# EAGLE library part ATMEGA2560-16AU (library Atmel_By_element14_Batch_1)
Microcontroller
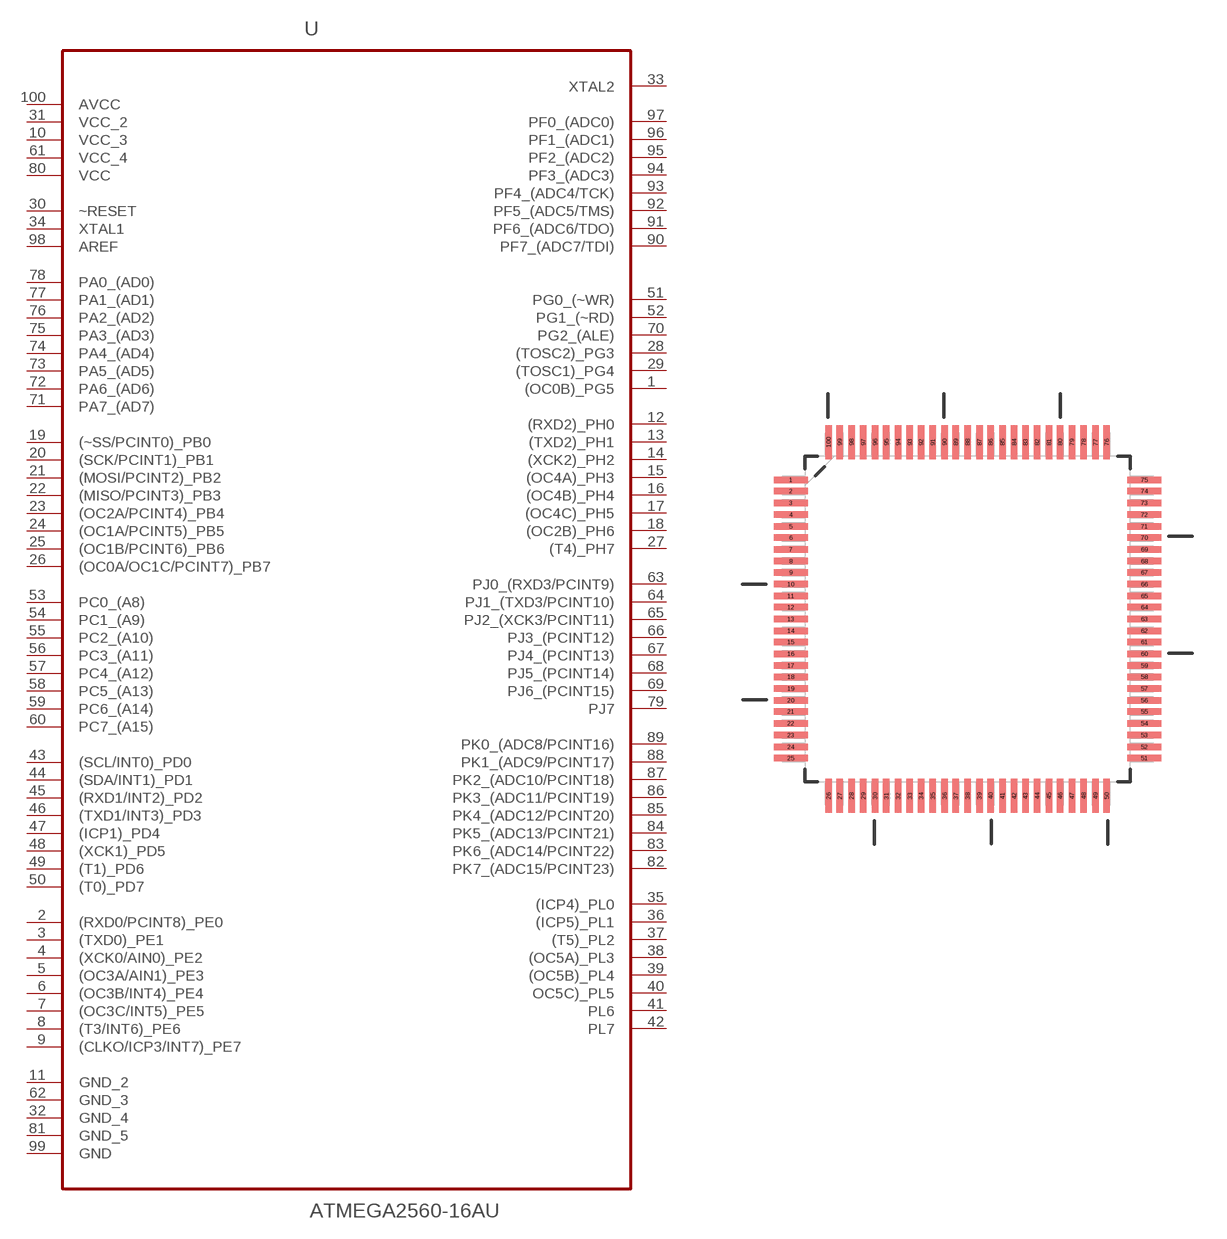
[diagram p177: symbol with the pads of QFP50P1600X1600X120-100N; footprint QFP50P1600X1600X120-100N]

Designator prefix U

## ATMEGA2560-16AU (DESCRIPTION: Microcontroller; MPN: ATMEGA2560-16AU; OC_FARNELL: 1288330; OC_NEWARK: 23M5051; PACKAGE: LQFP-100; SUPPLIER: ATMEL)  [QFP50P1600X1600X120-100N]
1  (OC0B)_PG5
2  (RXD0/PCINT8)_PE0
3  (TXD0)_PE1
4  (XCK0/AIN0)_PE2
5  (OC3A/AIN1)_PE3
6  (OC3B/INT4)_PE4
7  (OC3C/INT5)_PE5
8  (T3/INT6)_PE6
9  (CLKO/ICP3/INT7)_PE7
10  VCC_3  pwr
11  GND_2  pas
12  (RXD2)_PH0
13  (TXD2)_PH1
14  (XCK2)_PH2
15  (OC4A)_PH3
16  (OC4B)_PH4
17  (OC4C)_PH5
18  (OC2B)_PH6
19  (~SS/PCINT0)_PB0
20  (SCK/PCINT1)_PB1
21  (MOSI/PCINT2)_PB2
22  (MISO/PCINT3)_PB3
23  (OC2A/PCINT4)_PB4
24  (OC1A/PCINT5)_PB5
25  (OC1B/PCINT6)_PB6
26  (OC0A/OC1C/PCINT7)_PB7
27  (T4)_PH7
28  (TOSC2)_PG3
29  (TOSC1)_PG4
30  ~RESET  in
31  VCC_2  pwr
32  GND_4  pas
33  XTAL2  out
34  XTAL1  in
35  (ICP4)_PL0
36  (ICP5)_PL1
37  (T5)_PL2
38  (OC5A)_PL3
39  (OC5B)_PL4
40  OC5C)_PL5
41  PL6
42  PL7
43  (SCL/INT0)_PD0
44  (SDA/INT1)_PD1
45  (RXD1/INT2)_PD2
46  (TXD1/INT3)_PD3
47  (ICP1)_PD4
48  (XCK1)_PD5
49  (T1)_PD6
50  (T0)_PD7
51  PG0_(~WR)
52  PG1_(~RD)
53  PC0_(A8)
54  PC1_(A9)
55  PC2_(A10)
56  PC3_(A11)
57  PC4_(A12)
58  PC5_(A13)
59  PC6_(A14)
60  PC7_(A15)
61  VCC_4  pwr
62  GND_3  pas
63  PJ0_(RXD3/PCINT9)
64  PJ1_(TXD3/PCINT10)
65  PJ2_(XCK3/PCINT11)
66  PJ3_(PCINT12)
67  PJ4_(PCINT13)
68  PJ5_(PCINT14)
69  PJ6_(PCINT15)
70  PG2_(ALE)
71  PA7_(AD7)
72  PA6_(AD6)
73  PA5_(AD5)
74  PA4_(AD4)
75  PA3_(AD3)
76  PA2_(AD2)
77  PA1_(AD1)
78  PA0_(AD0)
79  PJ7
80  VCC  pwr
81  GND_5  pas
82  PK7_(ADC15/PCINT23)
83  PK6_(ADC14/PCINT22)
84  PK5_(ADC13/PCINT21)
85  PK4_(ADC12/PCINT20)
86  PK3_(ADC11/PCINT19)
87  PK2_(ADC10/PCINT18)
88  PK1_(ADC9/PCINT17)
89  PK0_(ADC8/PCINT16)
90  PF7_(ADC7/TDI)
91  PF6_(ADC6/TDO)
92  PF5_(ADC5/TMS)
93  PF4_(ADC4/TCK)
94  PF3_(ADC3)
95  PF2_(ADC2)
96  PF1_(ADC1)
97  PF0_(ADC0)
98  AREF  in
99  GND  pas
100  AVCC  pwr

## Footprint QFP50P1600X1600X120-100N (pad centres in mm)
smd 1.473 x 0.279: 1 -7.62,5.994; 2 -7.62,5.512; 3 -7.62,5.004; 4 -7.62,4.496; 5 -7.62,3.988; 6 -7.62,3.505; 7 -7.62,2.997; 8 -7.62,2.489; 9 -7.62,2.007; 10 -7.62,1.499; 11 -7.62,0.991; 12 -7.62,0.508; 13 -7.62,0; 14 -7.62,-0.508; 15 -7.62,-0.991; 16 -7.62,-1.499; 17 -7.62,-2.007; 18 -7.62,-2.489; 19 -7.62,-2.997; 20 -7.62,-3.505; 21 -7.62,-3.988; 22 -7.62,-4.496; 23 -7.62,-5.004; 24 -7.62,-5.512; 25 -7.62,-5.994; 51 7.62,-5.994; 52 7.62,-5.512; 53 7.62,-5.004; 54 7.62,-4.496; 55 7.62,-3.988; 56 7.62,-3.505; 57 7.62,-2.997; 58 7.62,-2.489; 59 7.62,-2.007; 60 7.62,-1.499; 61 7.62,-0.991; 62 7.62,-0.508; 63 7.62,0; 64 7.62,0.508; 65 7.62,0.991; 66 7.62,1.499; 67 7.62,2.007; 68 7.62,2.489; 69 7.62,2.997; 70 7.62,3.505; 71 7.62,3.988; 72 7.62,4.496; 73 7.62,5.004; 74 7.62,5.512; 75 7.62,5.994
smd 0.279 x 1.473: 26 -5.994,-7.62; 27 -5.512,-7.62; 28 -5.004,-7.62; 29 -4.496,-7.62; 30 -3.988,-7.62; 31 -3.505,-7.62; 32 -2.997,-7.62; 33 -2.489,-7.62; 34 -2.007,-7.62; 35 -1.499,-7.62; 36 -0.991,-7.62; 37 -0.508,-7.62; 38 0,-7.62; 39 0.508,-7.62; 40 0.991,-7.62; 41 1.499,-7.62; 42 2.007,-7.62; 43 2.489,-7.62; 44 2.997,-7.62; 45 3.505,-7.62; 46 3.988,-7.62; 47 4.496,-7.62; 48 5.004,-7.62; 49 5.512,-7.62; 50 5.994,-7.62; 76 5.994,7.62; 77 5.512,7.62; 78 5.004,7.62; 79 4.496,7.62; 80 3.988,7.62; 81 3.505,7.62; 82 2.997,7.62; 83 2.489,7.62; 84 2.007,7.62; 85 1.499,7.62; 86 0.991,7.62; 87 0.508,7.62; 88 0,7.62; 89 -0.508,7.62; 90 -0.991,7.62; 91 -1.499,7.62; 92 -2.007,7.62; 93 -2.489,7.62; 94 -2.997,7.62; 95 -3.505,7.62; 96 -3.988,7.62; 97 -4.496,7.62; 98 -5.004,7.62; 99 -5.512,7.62; 100 -5.994,7.62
